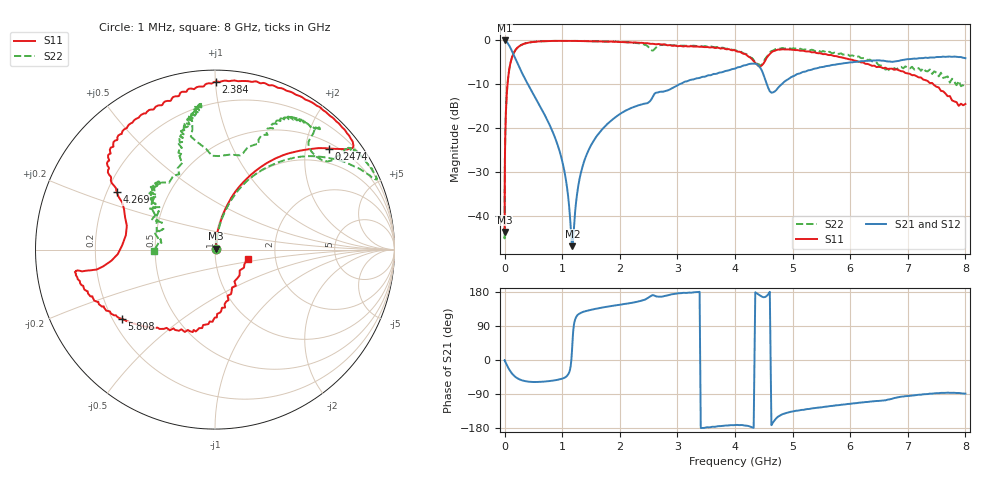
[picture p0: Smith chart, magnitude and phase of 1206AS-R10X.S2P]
!s-Parameter Generated by FASTRON Sdn. Bhd.
!FASTRON P/N : 1206AS-R10X
!Keysight Technologies: E5071C_MY46733604_B.14.02
!Date: Wed Nov 15 10:57:56 2023
!Version  :Rev00  Wed Nov 15 10:57:56 2023
!Data & Calibration Information:
!Freq  S11:SOLT2(ON)  S21:SOLT2(ON)  S12:SOLT2(ON)  S22:SOLT2(ON)
!PortZ  Port1:50+j0  Port2:50+j0
!When reading reference impedance value at option line is always used.
! Remarks : This data is being provided solely for informational purposes.
# Hz S dB R 50
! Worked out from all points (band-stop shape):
!   1601 points, 1 MHz to 8 GHz, reference 50 ohm
!   highest |S21| = -0.03 dB at 1.486 MHz (marker M1); lowest = -46.8 dB at 1.179 GHz (marker M2)
!   |S21| within 3 dB of the highest: start of sweep to 148.7 MHz
!   lowest |S11| = -43.6 dB at 1.053 MHz (marker M3), VSWR 1.01, Z = 50.5 + j0.439 ohm
!   |S11| at or under -10 dB: start of sweep to 51.12 MHz; 7.444 GHz to end of sweep
!   |S22| runs from -45.0 to -0.1 dB; largest |S21 - S12| = 0.0074
!   S11 on the Smith chart (normalised r, x): 1 MHz: 1.01, +0.01; 247.4 MHz: 0.62, +2.50; 2.384 GHz: 0.07, +1.00; 4.269 GHz: 0.24, +0.26; 5.808 GHz: 0.24, -0.31; 8 GHz: 1.43, -0.16
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1000000  -42.89 35.7  -0.04 -0.5  -0.05 -0.4  -43.74 42.6
1052806  -43.57 41.0  -0.04 -0.5  -0.06 -0.4  -44.04 40.0
1486461  -40.52 59.6  -0.03 -0.6  -0.05 -0.6  -41.06 51.0
4479405  -30.26 77.9  -0.06 -1.6  -0.06 -1.6  -30.33 79.3
2.00676e7  -17.60 79.9  -0.15 -7.0  -0.16 -6.9  -17.56 79.2
8.994653e7  -5.96 62.2  -1.41 -27.3  -1.41 -27.3  -5.97 60.2
2.474433e8  -1.42 41.5  -5.90 -50.3  -5.91 -50.3  -1.41 35.9
4.006501e8  -0.56 36.8  -9.88 -56.9  -9.88 -56.9  -0.56 27.5
8.843521e8  -0.15 44.0  -22.41 -53.3  -22.42 -53.3  -0.13 23.9
1.030344e9  -0.13 48.2  -29.17 -47.5  -29.17 -47.5  -0.14 24.8
1.14826e9  -0.15 51.7  -42.51 -15.8  -42.51 -15.9  -0.15 25.7
1.179402e9  -0.14 52.6  -46.77 48.0  -46.83 47.9  -0.15 26.2
1.380485e9  -0.21 58.7  -27.54 127.8  -27.56 127.7  -0.14 28.0
1.7949e9  -0.32 71.7  -18.88 140.8  -18.91 140.6  -0.29 32.5
2.384191e9  -0.58 89.8  -14.56 157.0  -14.60 156.8  -0.79 37.7
3.466968e9  -1.55 125.8  -8.28 -179.2  -8.31 -179.2  -1.34 57.6
4.26866e9  -3.95 149.7  -5.33 -176.0  -5.31 -176.0  -3.90 67.5
4.632554e9  -2.74 -170.7  -11.90 -172.0  -11.87 -172.1  -2.45 101.1
4.912472e9  -2.07 -169.7  -8.93 -138.9  -8.89 -139.1  -1.77 95.4
5.808211e9  -3.80 -143.3  -5.37 -119.0  -5.35 -119.4  -3.06 102.4
6.920464e9  -7.07 -99.3  -4.46 -96.3  -4.44 -97.0  -6.35 131.3
8e9  -14.47 -16.0  -4.06 -88.8  -4.04 -89.3  -9.42 -179.1
